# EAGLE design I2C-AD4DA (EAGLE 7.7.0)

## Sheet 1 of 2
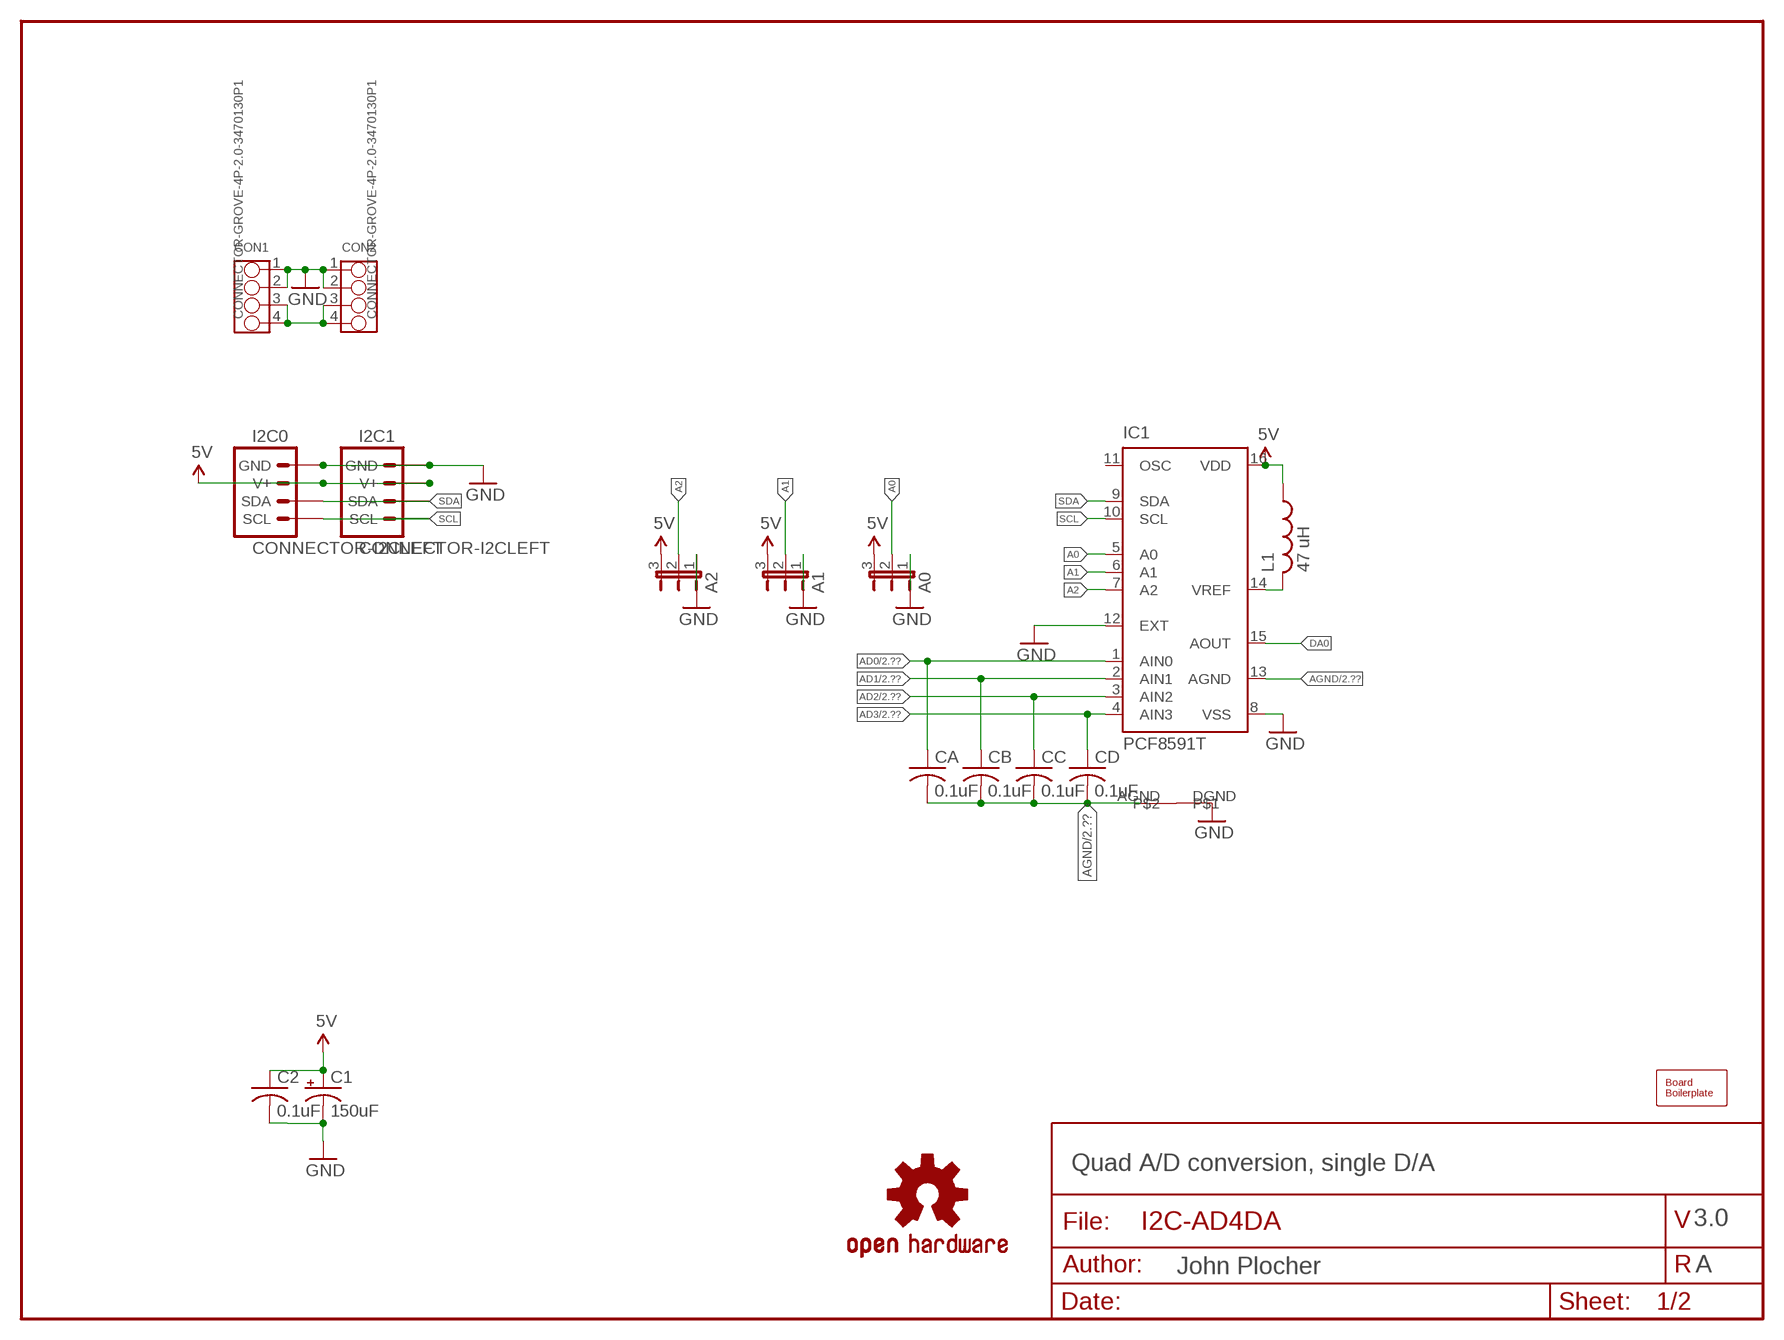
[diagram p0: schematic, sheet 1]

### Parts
A0  JUMPER-31-2  [SJ_3_PASTE1&2]
A1  JUMPER-31-2  [SJ_3_PASTE1&2]
A2  JUMPER-31-2  [SJ_3_PASTE1&2]
BOARD1  BOARD80X100  [BOARD-DINRAIL-3.17INX10CM]
C1  150uF  CAP-POLUD10X10  [UD-10X10_NICHICON]
C2  0.1uF  CAP0805  [0805-CAP]
CA  0.1uF  CAP0805  [0805-CAP]
CB  0.1uF  CAP0805  [0805-CAP]
CC  0.1uF  CAP0805  [0805-CAP]
CD  0.1uF  CAP0805  [0805-CAP]
CON1  CONNECTOR-GROVE-4P-2.0-3470130P1  [4P-2.0]
CON2  CONNECTOR-GROVE-4P-2.0-3470130P1  [4P-2.0]
I2C0  CONNECTOR-I2CLEFT  [I2C-L]
I2C1  CONNECTOR-I2CLEFT  [I2C-L]
IC1  PCF8591T  [SO16W]
L1  47 uH  L-USL2012C  [L2012C]
LOGO1  DOC-OSHW-LOGO-L  [OSHW-LOGO-L]
U$1  AGND+DGND  [AGND+DGND]

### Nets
5V: A0.3 A1.3 A2.3 C1.+ C2.1 I2C0.V+ I2C0.V+@1(V+) I2C1.V+ I2C1.V+@1(V+) IC1.16(VDD) L1.1 ; also sheet 2
A0: A0.2 IC1.5(A0)
A1: A1.2 IC1.6(A1)
A2: A2.2 IC1.7(A2)
AD0: CA.1 IC1.1(AIN0) ; also sheet 2
AD1: CB.1 IC1.2(AIN1) ; also sheet 2
AD2: CC.1 IC1.3(AIN2) ; also sheet 2
AD3: CD.1 IC1.4(AIN3) ; also sheet 2
AGND: CA.2 CB.2 CC.2 CD.2 IC1.13(AGND) U$1.AGND ; also sheet 2
DA0: IC1.15(AOUT)
GND: A0.1 A1.1 A2.1 C1.- C2.2 CON1.1 CON1.2 CON2.1 CON2.2 I2C0.GND I2C0.GND@1(GND) I2C1.GND I2C1.GND@1(GND) IC1.8(VSS) IC1.12(EXT) U$1.DGND ; also sheet 2
N$1: IC1.14(VREF) L1.2
SCL: I2C0.SCL I2C0.SCL@1(SCL) I2C1.SCL I2C1.SCL@1(SCL) IC1.10(SCL)
SDA: I2C0.SDA I2C0.SDA@1(SDA) I2C1.SDA I2C1.SDA@1(SDA) IC1.9(SDA)
VIN: CON1.3 CON1.4 CON2.3 CON2.4
Unconnected: IC1.11(OSC)

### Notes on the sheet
- Quad A/D conversion, single D/A
- 3.0
- A

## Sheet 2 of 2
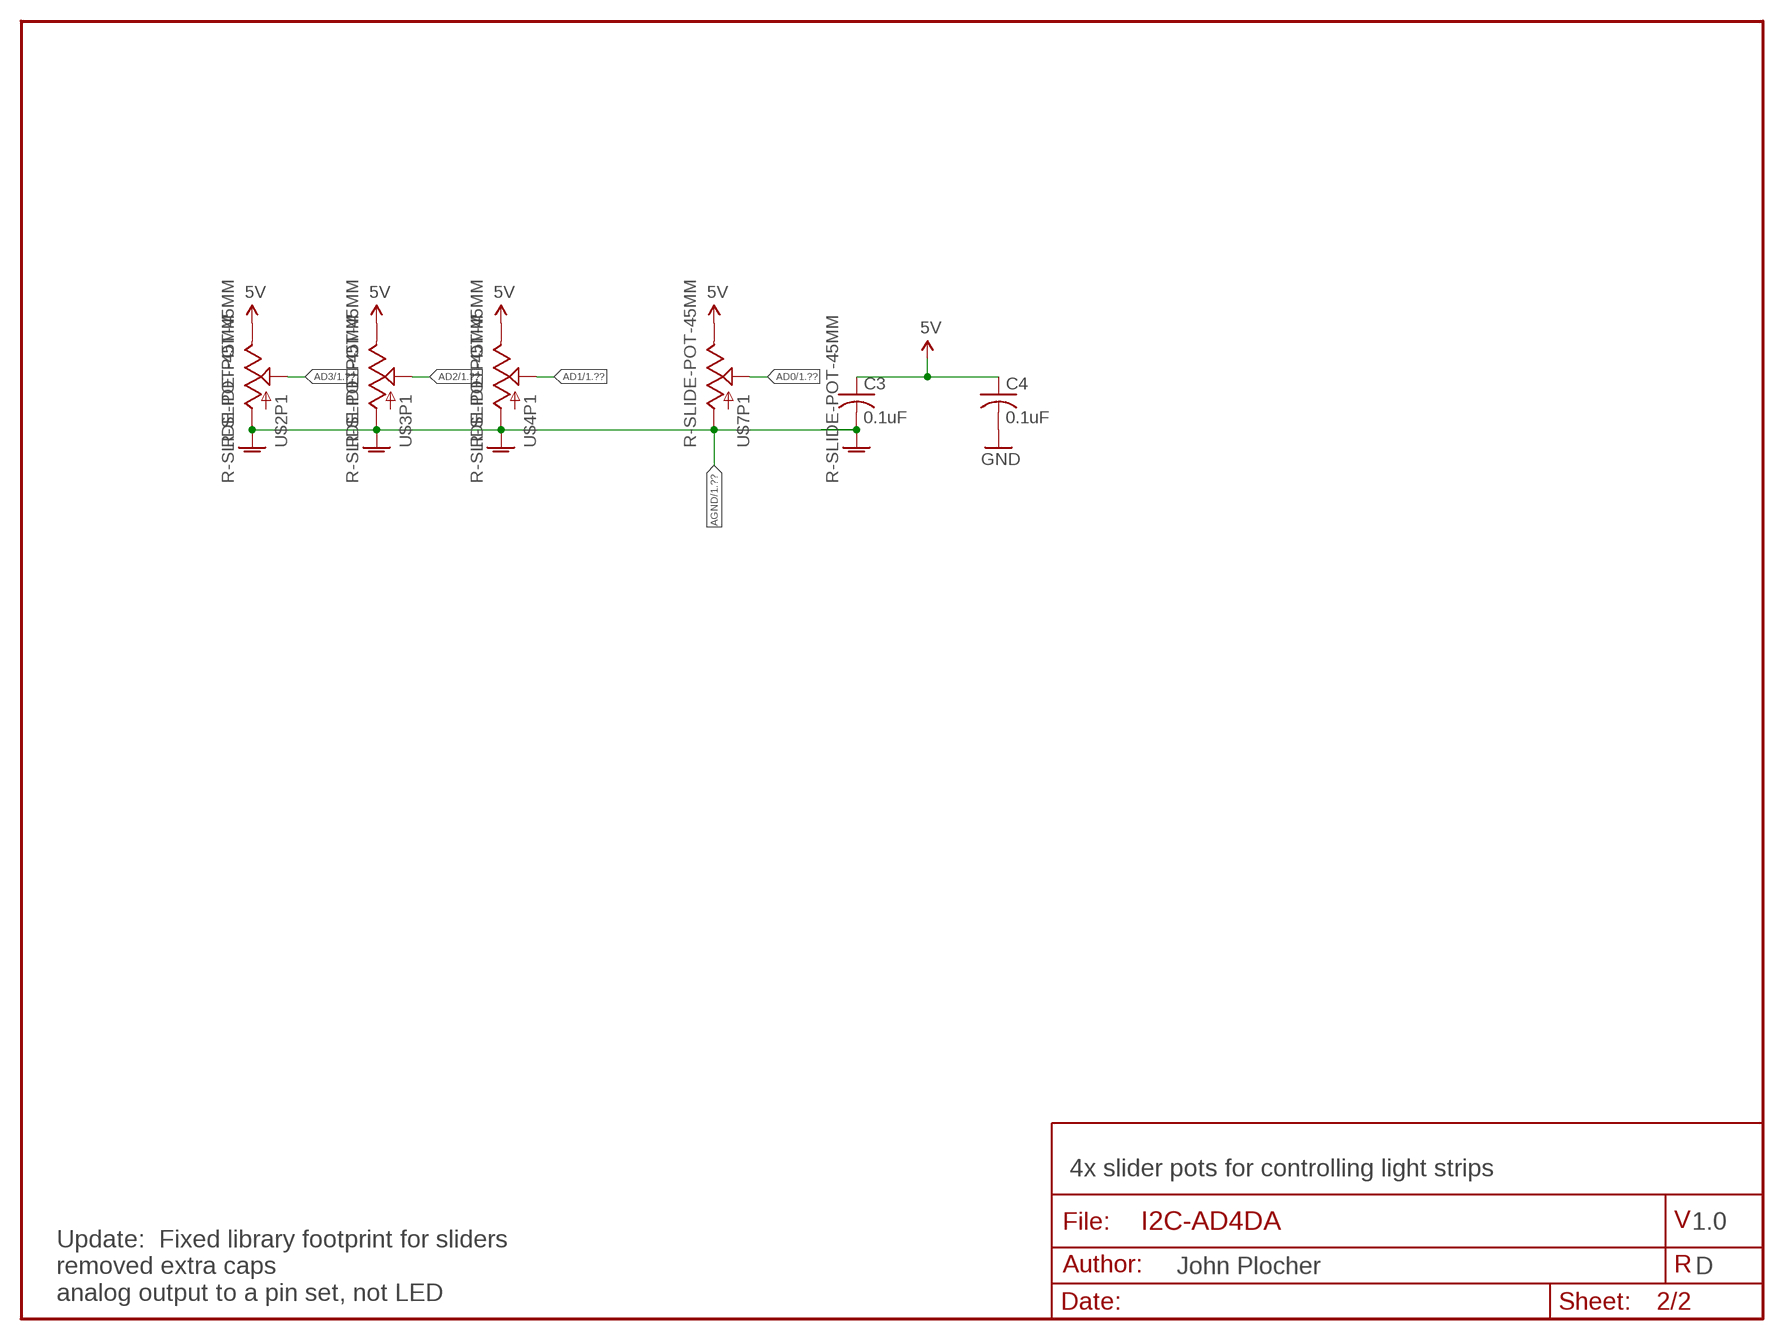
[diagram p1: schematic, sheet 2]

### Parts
C3  0.1uF  CAP0805  [0805-CAP]
C4  0.1uF  CAP0805  [0805-CAP]
U$2  R-SLIDE-POT-45MM  [SLIDER-45MM]
U$3  R-SLIDE-POT-45MM  [SLIDER-45MM]
U$4  R-SLIDE-POT-45MM  [SLIDER-45MM]
U$7  R-SLIDE-POT-45MM  [SLIDER-45MM]

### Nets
5V: C3.1 C4.1 U$2.E(P1:E) U$3.E(P1:E) U$4.E(P1:E) U$7.E(P1:E) ; also sheet 1
AD0: U$7.S(P1:S) ; also sheet 1
AD1: U$4.S(P1:S) ; also sheet 1
AD2: U$3.S(P1:S) ; also sheet 1
AD3: U$2.S(P1:S) ; also sheet 1
AGND: C3.2 U$2.A(P1:A) U$2.AGND@0(AGND) U$2.AGND@1(AGND) U$3.A(P1:A) U$3.AGND@0(AGND) U$3.AGND@1(AGND) U$4.A(P1:A) U$4.AGND@0(AGND) U$4.AGND@1(AGND) U$7.A(P1:A) U$7.AGND@0(AGND) U$7.AGND@1(AGND) ; also sheet 1
GND: C4.2 ; also sheet 1

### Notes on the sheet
- 4x slider pots for controlling light strips
- 1.0
- D
- Update:  Fixed library footprint for sliders
  removed extra caps
  analog output to a pin set, not LED

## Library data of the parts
A0 A1 A2 = SPCoast:JUMPER-3
BOARD1 = SPCoast:BOARD
C1 = SPCoast:CAP-POL*
C2-C4 CA CB CC CD = SPCoast:CAP*
CON1 CON2 = SPCoast:CONNECTOR-GROVE-4P-2.0
I2C0 I2C1 = SPCoast:CONNECTOR-I2C
IC1 = SPCoast:PCF8591: I2C-Bus D/A CONVERTER; MPN: PCF8591T/2,512; OC_FARNELL: 1826767; OC_NEWARK: 70R6911
L1 = SPCoast:L-US: INDUCTOR, American symbol
LOGO1 = SPCoast:DOC-OSHW-LOGO-: Open Source Hardware Logo
U$1 = SPCoast:AGND+DGND
U$2-U$4 U$7 = SPCoast:R-SLIDE-POT: Slide-type potentiometer- COM-9119

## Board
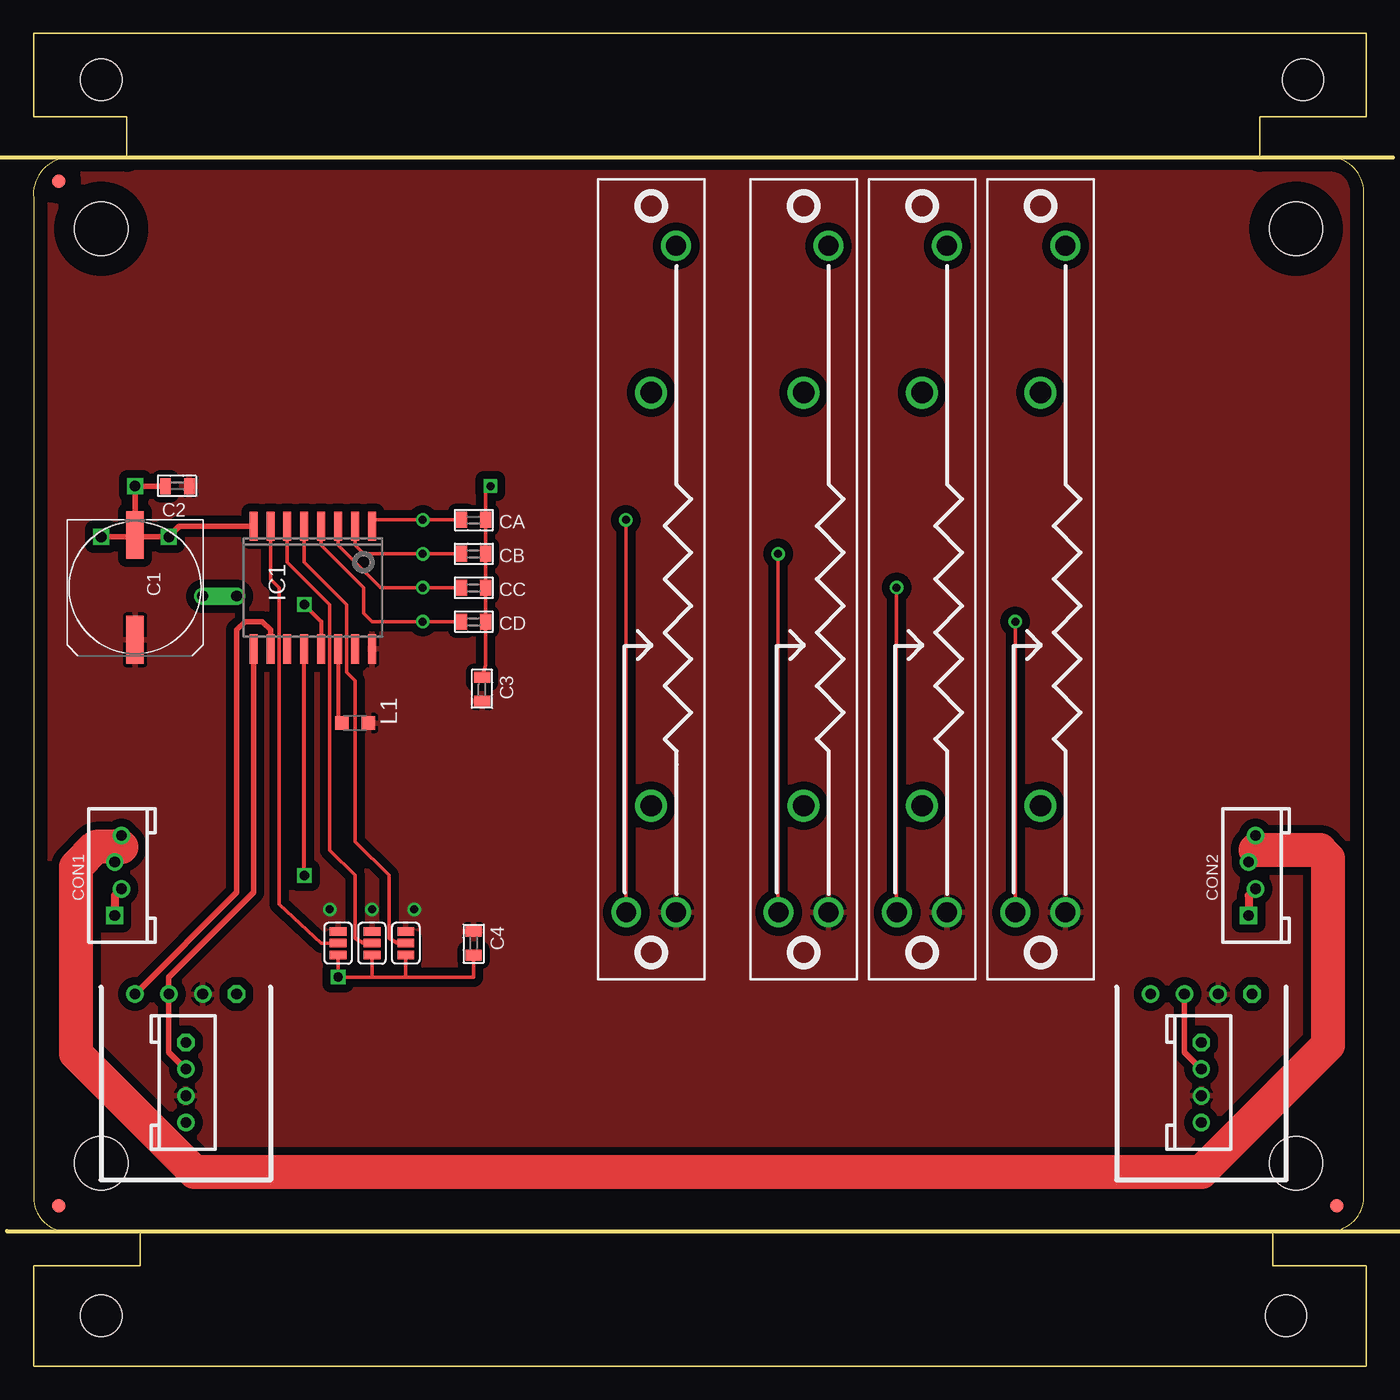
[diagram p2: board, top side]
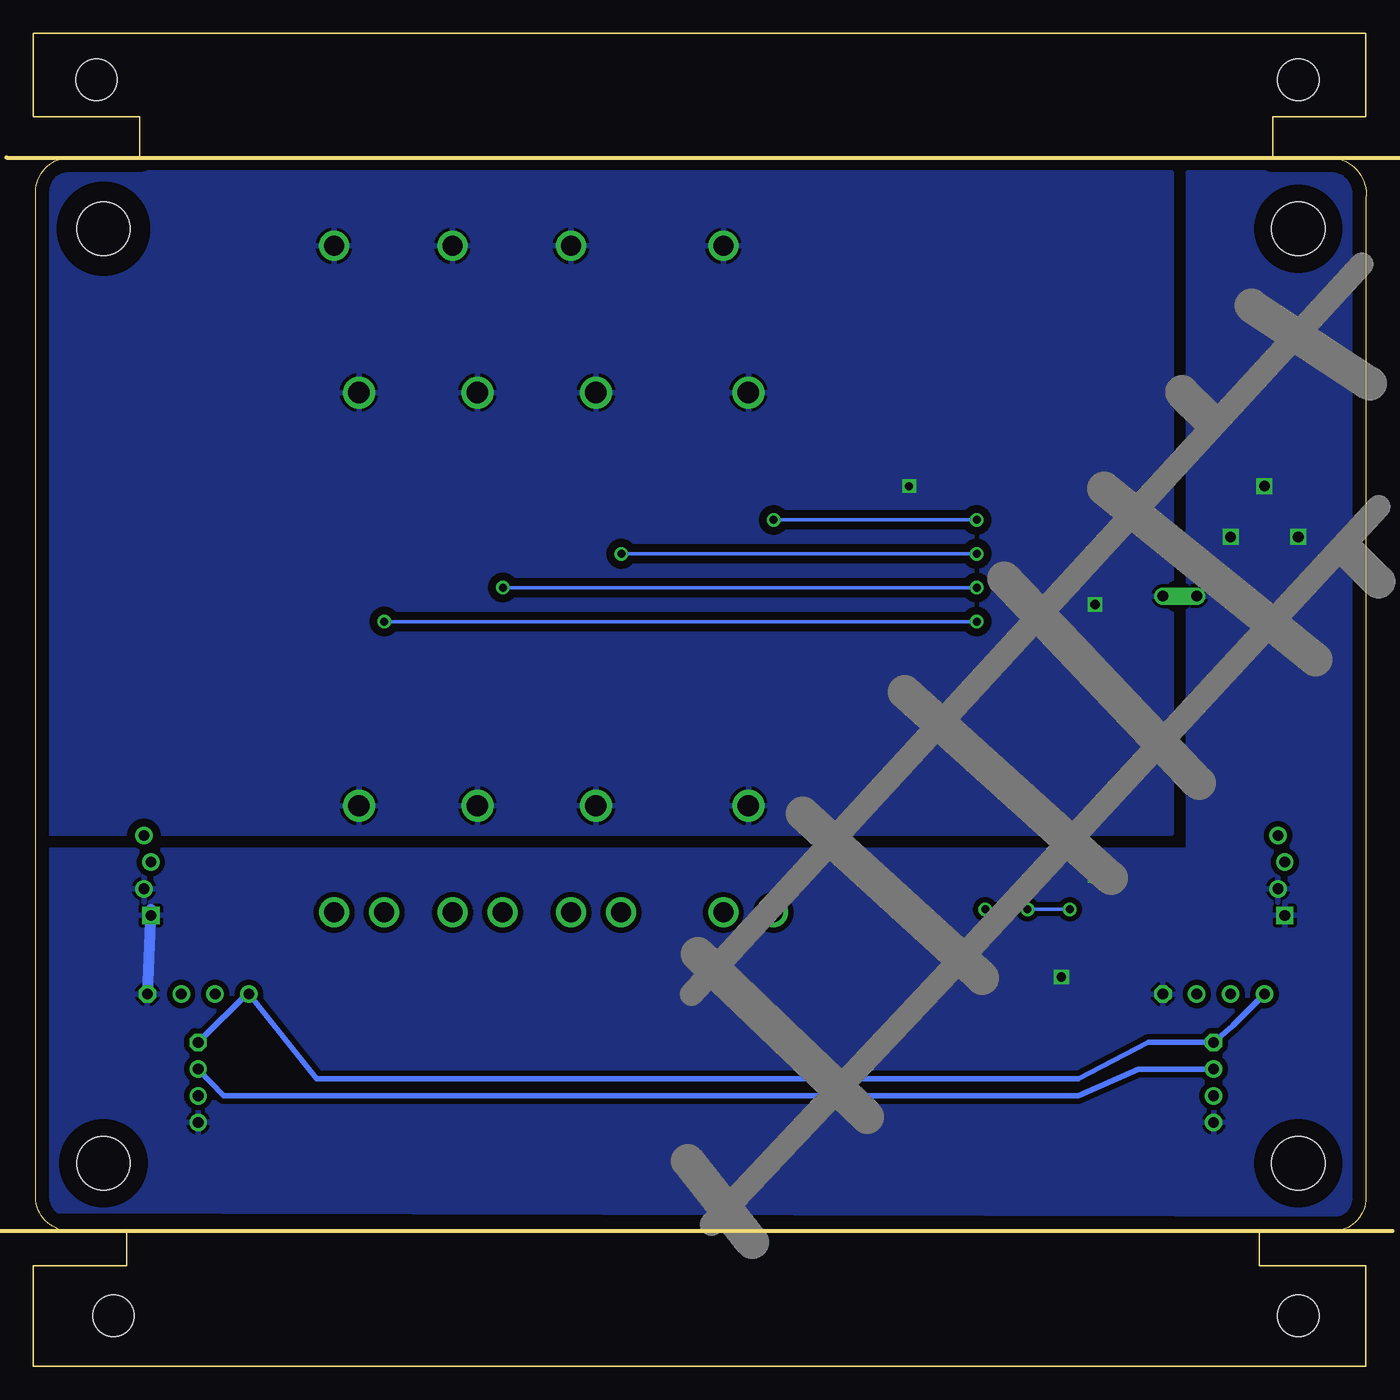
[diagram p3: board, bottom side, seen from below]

Size 100.01 x 100 mm. Coordinates in mm from the lower left corner, seen from the top.
Copper layers (1*16): Top 0.035mm / dielectric 1.5mm / Bottom 0.035mm
Design rules "default": minimum track width 10mil, minimum drill 0.6mm, track to track 8mil, track to pad 8mil, pad to pad 8mil, via to via 8mil, smd to smd 8mil, copper to edge 40mil, drill to drill 8mil, minimum pad ring 10mil, minimum via ring 8mil, stop-mask expansion 4mil, vias tented up to drill 0mil, thermal gap 10mil

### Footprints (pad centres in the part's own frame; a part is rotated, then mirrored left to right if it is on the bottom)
SJ_3_PASTE1&2 = smd 0.635 x 1.27: 1 -0.889,0; 2 0,0; 3 0.889,0
BOARD-DINRAIL-3.17INX10CM = smd 1 x 1: 1 1.905,12.065; 2 97.79,12.065; 3 1.905,88.9 | hole 4: 94.742,15.24; 5.08,85.344; 94.742,85.344; 5.08,15.24 | hole 3.1: 5.08,96.52; 95.25,96.52; 5.08,3.81; 93.98,3.81
UD-10X10_NICHICON = smd 3.6 x 1.3: + 3.925,0; - -3.95,0
0805-CAP = smd 0.8 x 1.2: 1 -0.9,0; 2 0.9,0
4P-2.0 = drill 0.8 pad 1.27 square: 1 -3,0.254 | drill 0.8 pad 1.27: 2 -1,-0.254; 3 1,0.254; 4 3,-0.254
I2C-L = drill 0.8 octagon: GND 3.81,0 | drill 0.8 pad 1.27: GND@1 0,-9.635; SDA@1 0,-5.635; V+@1 0,-7.635 | drill 0.8: SCL -3.81,0; SDA -1.27,0; V+ 1.27,0 | drill 0.8 pad 1.27 octagon: SCL@1 0,-3.635
SO16W = smd 0.6 x 2.2: 1 -4.445,-4.6; 2 -3.175,-4.6; 3 -1.905,-4.6; 4 -0.635,-4.6; 5 0.635,-4.6; 6 1.905,-4.6; 7 3.175,-4.6; 8 4.445,-4.6; 9 4.445,4.6; 10 3.175,4.6; 11 1.905,4.6; 12 0.635,4.6; 13 -0.635,4.6; 14 -1.905,4.6; 15 -3.175,4.6; 16 -4.445,4.6
L2012C = smd 1 x 1: 1 -1,0; 2 1,0
AGND+DGND = drill 0.8 offset: AGND -1.27,0; DGND 1.27,0
SLIDER-45MM = drill 1.5: A 25,-1.875; E -25,-1.875; S -25,1.875 | drill 1.6: AGND@0 -17,0; AGND@1 14,0

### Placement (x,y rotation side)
A0  27.95,31.75 90 top
A1  25.41,31.75 90 top
A2  22.87,31.75 90 top
BOARD1  0.01,0 0 top
C1  7.63,58.42 270 top
C2  10.81,66.04 180 top
C3  33.67,50.8 90 top
C4  33.03,31.75 270 top
CA  33.03,63.5 0 top
CB  33.03,60.96 0 top
CC  33.03,58.42 0 top
CD  33.03,55.88 0 top
CON1  6.36,36.83 90 top
CON2  91.45,36.83 90 top
I2C0  11.44,27.94 0 top
I2C1  87.64,27.94 0 top
IC1  20.97,58.42 180 top
L1  24.14,48.26 180 top
LOGO1  7.63,77.47 0 top
U$1  13.98,57.78 180 top
U$2  75.58,59.05 90 top
U$3  66.69,59.05 90 top
U$4  57.8,59.05 90 top
U$7  46.37,59.05 90 top

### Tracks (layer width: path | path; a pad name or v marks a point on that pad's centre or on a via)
5V  (via drill 0.6)
  Bottom 0.254: v22.24,34.29 v25.41,34.29 v28.59,34.29
  pour Top (isolate 0.61): 0.01,89.53 100.01,89.53 100.01,9.79 0.01,9.53
A0
  Top 0.254: IC1.5 20.33,60.33 23.51,57.15 23.51,52.07 24.14,51.44 24.14,39.37 26.68,36.83 26.68,32.13 27.32,31.75 A0.2
A1
  Top 0.254: IC1.6 19.06,60.33 22.24,57.15 22.24,38.73 24.14,36.83 24.14,32.13 24.78,31.75 A1.2
A2
  Top 0.254: IC1.7 17.79,59.05 18.43,58.42 18.43,34.67 21.6,31.75 A2.2
AD0  (via drill 0.6)
  Top 0.254: CA.1 v29.22,63.5 25.41,63.5 IC1.1 | v44.46,63.5 44.46,34.09 U$7.S
  Bottom 0.254: v29.22,63.5 v44.46,63.5
AD1  (via drill 0.6)
  Top 0.254: CB.1 v29.22,60.96 24.78,60.96 24.14,61.59 IC1.2 | v55.89,60.96 55.89,34.09 U$4.S
  Bottom 0.254: v29.22,60.96 v55.89,60.96
AD2  (via drill 0.6)
  Top 0.254: CC.1 v29.22,58.42 26.05,58.42 22.87,61.59 IC1.3 | v64.78,58.42 64.78,34.09 U$3.S
  Bottom 0.254: v29.22,58.42 v64.78,58.42
AD3  (via drill 0.6)
  Top 0.254: CD.1 v29.22,55.88 25.41,55.88 24.78,56.52 24.78,58.42 21.6,61.59 IC1.4 | v73.67,55.88 73.67,34.09 U$2.S
  Bottom 0.254: v29.22,55.88 v73.67,55.88
AGND  (via drill 0.6, 0.7)
  Top 0.254: v34.3,66.04 33.93,65.67 CA.2 CB.2 CC.2 CD.2 33.93,52.6 C3.2
  Top 0.305: IC1.13 21.6,55.88 v20.33,57.15
  pour Bottom (isolate 0.61): 14.62,40.01 14.62,89.53 99.84,89.53 99.84,40.01
GND  (via drill 0.7, 0.8)
  Top 0.254: A2.1 v22.87,29.21 25.41,29.21 | A1.1 25.41,29.21 | A0.1 27.95,29.21 | 27.95,29.21 25.41,29.21 | C4.2 33.03,29.21 27.95,29.21
  Top 0.305: v20.33,36.83 IC1.12
  Top 0.406: 16.52,63.5 IC1.8 10.96,63.02 v10.17,62.23 7.63,62.23 v7.63,66.04 C2.2 | v5.09,62.23 7.49,62.23 C1.-
  Top 0.61: CON1.2 6.11,35.32 CON1.1 | CON2.2 91.2,35.32 CON2.1
  Bottom 0.813: CON2.1 91.2,34.29 I2C1.GND
  pour Bottom (isolate 0.406): 0.01,89.53 13.35,89.53 13.35,38.73 100.19,38.73 100.19,11.7 0.01,11.43
N$1
  Top 0.305: IC1.14 22.87,48.53 L1.2
SCL
  Top 0.406: IC1.10 17.79,55.24 17.16,55.88 15.89,55.88 15.25,55.24 15.25,35.56 I2C0.SCL
  Bottom 0.406: I2C0.SCL 10,25.57 I2C0.SCL@1 16.35,24.3 21.6,21.59 78.75,21.59 I2C1.SCL 83.83,28.11 I2C1.SCL@1
SDA
  Top 0.406: I2C0.SDA@1 10.17,23.57 I2C0.SDA 10.17,29.21 16.52,35.56 IC1.9 | I2C1.SDA 86.37,23.57 I2C1.SDA@1
  Bottom 0.406: I2C0.SDA@1 17.08,22.3 21.6,20.32 85.74,20.32 I2C1.SDA@1
VIN
  Top 0.61: CON1.3 6.62,38.97 CON1.4 | CON2.3 91.71,38.34 91.71,38.73 CON2.4
  Top 2.54: 6.62,38.97 4.7,38.97 3.19,37.47 3.19,23.5 12.08,14.61 87.64,14.61 97.17,24.13 97.17,38.1 96.53,38.73 91.71,38.73

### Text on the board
tDocu: v3.0 | 2019-04 | OSHW | John Plocher | LightUI | I2C-AD4DA | Vin | Vin | 5v | 5v | 0 1 | AD0 | AD1 | AD2 | AD3 | Board / Address | W | R G B | LightUI | I2C-AD4DA
bDocu: Solder Side | Made in the PCR, Coast Division, NMRA | AD4DA | Go Bears! | Model Railroading is fun! | LightUI | www . SPCoast . com | I2C / Address | A2 A1 A0 | *B0: 0 0 0 0x48 | B1: 0 0 1 0x49 | B2: 0 1 0 0x4A | B3: 0 1 1 0x4B | B4: 1 0 0 0x4C | Board / Address | B5: 1 0 1 0x4D | B6: 1 1 0 0x4E | B7: 1 1 1 0x3F

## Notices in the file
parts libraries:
SparkFun-Aesthetics: Licensing: CC v3.0 Share-Alike You are welcome to use this library for commercial purposes.
SPCoast: http://freedomdefined.org/OSHW Creative Commons - Attribution - ShareAlike 3.0
